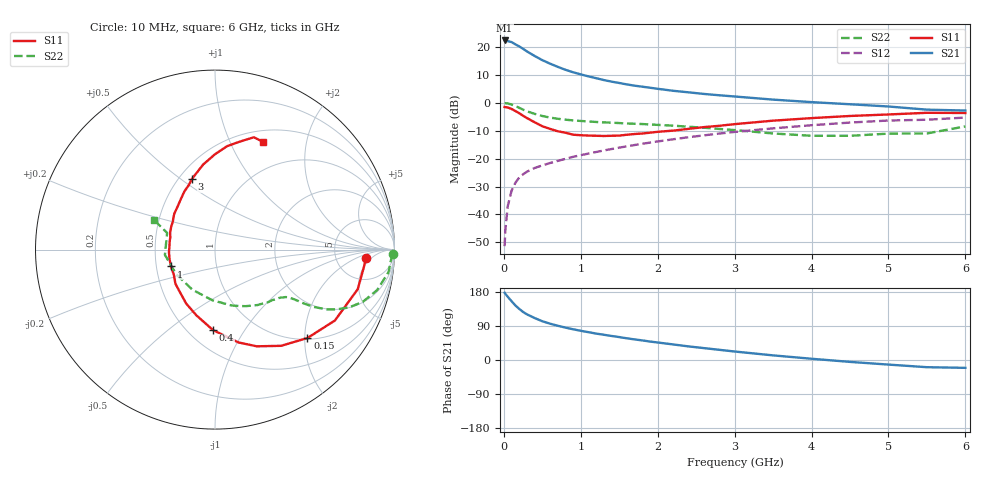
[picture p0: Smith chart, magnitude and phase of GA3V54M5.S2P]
! Infineon Technologies  Discrete & RF Semiconductors
! BF775
! Si NPN RF Bipolar Junction Transistor in SOT23
! VCE = 3.5 V  IC = 4.5 mA
! Common Emitter S-Parameters:  May  1996
# GHz  S  MA  R  50
!  f  S11  S21  S12  S22
! GHz  MAG  ANG  MAG  ANG  MAG  ANG  MAG  ANG
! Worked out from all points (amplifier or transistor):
!   36 points, 10 MHz to 6 GHz, reference 50 ohm
!   highest |S21| = 22.3 dB at 10 MHz (marker M1)
!   |S21| within 3 dB of that: start of sweep to 250.5 MHz
!   unconditionally stable (mu >= 1): 835.6 MHz to 3.478 GHz
!   at 250 MHz: K = 0.46, MSG = 22.5 dB, |S12| = -25.6 dB
!   at 1.4 GHz: K = 1.12, MAG = 9.9 dB, |S12| = -16.6 dB
!   at 6 GHz: K = 0.96, MSG = 1.3 dB, |S12| = -5.3 dB
!   S11 on the Smith chart (normalised r, x): 10 MHz: 10, -3; 150 MHz: 1.03, -2.06; 400 MHz: 0.65, -0.73; 1 GHz: 0.60, -0.12; 3 GHz: 0.58, +0.55; 6 GHz: 0.64, +1.34
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0.01  0.8401 -3.3  13.1 177.5  0.0027 89.1  0.9931 -1.4
0.02  0.8359 -6.4  12.88 174.6  0.0053 85.5  0.9835 -2.9
0.05  0.8253 -15.5  12.76 167.1  0.0139 81.1  0.9751 -7.4
0.1  0.7761 -30.6  12.26 155.2  0.0265 74.2  0.9313 -14.0
0.15  0.7128 -43.7  11.15 143.9  0.0369 68.2  0.8739 -19.4
0.2  0.6505 -55.5  10.25 134.9  0.0458 63.8  0.8141 -23.3
0.25  0.5866 -66.7  9.283 126.8  0.0523 60.1  0.7546 -26.2
0.3  0.5336 -75.8  8.342 120.5  0.0583 58.0  0.7051 -28.2
0.4  0.4486 -91.4  6.91 110.8  0.0679 55.2  0.634 -30.2
0.5  0.3807 -105.8  5.814 102.3  0.0756 54.7  0.5803 -31.2
0.6  0.3411 -118.0  5.037 95.9  0.0833 55.0  0.5438 -31.7
0.8  0.291 -139.3  3.91 85.5  0.0989 55.2  0.4983 -32.7
1  0.2627 -159.0  3.231 77.1  0.1151 55.8  0.473 -34.0
1.1  0.2587 -168.1  2.977 73.4  0.1232 56.2  0.4636 -35.1
1.3  0.2543 176.5  2.557 66.6  0.1401 56.2  0.4464 -37.2
1.6  0.2681 158.8  2.135 57.2  0.1664 55.7  0.4259 -41.3
2.2  0.3174 131.1  1.643 41.1  0.222 52.4  0.3897 -52.4
3  0.4148 108.0  1.298 22.4  0.3009 45.3  0.3244 -73.6
3.5  0.4786 97.9  1.141 12.2  0.3485 39.6  0.2824 -93.1
4.5  0.5811 83.2  0.942 -5.0  0.4426 26.8  0.2563 -147.6
5.5  0.6624 70.9  0.754 -19.0  0.4975 11.6  0.2824 160.8
6  0.657 65.8  0.727 -20.7  0.5441 7.4  0.3782 154.0
